FUNCTION FC 80 : VOID
TITLE =BLOCK FOR BALANCING PRESS
AUTHOR : Esposito
FAMILY : EGAL_srl
NAME : BALANCIN
VERSION : 0.1


VAR_TEMP
  VALUE_TONN : REAL ;	//Value in tonn of the weight slide addition die
  VALUE_BAR : REAL ;	//Value in Bar of the cylinders balancing slide
  OFF_SET_LOAD : REAL ;	//Value in Bar of the OFF SET for load valve balancing
  OFF_SET_DISC : REAL ;	//Value in Bar of the OFF SET for discarge valve balancing
  OFF_SET_LOAD_H : REAL ;
  OFF_SET_DISC_L : REAL ;
  TON_VIS_OP37 : REAL ;
  MIN_MAX_VAL_OP37 : REAL ;
END_VAR
BEGIN
NETWORK
TITLE =CONDITIONS FOR BALANCING
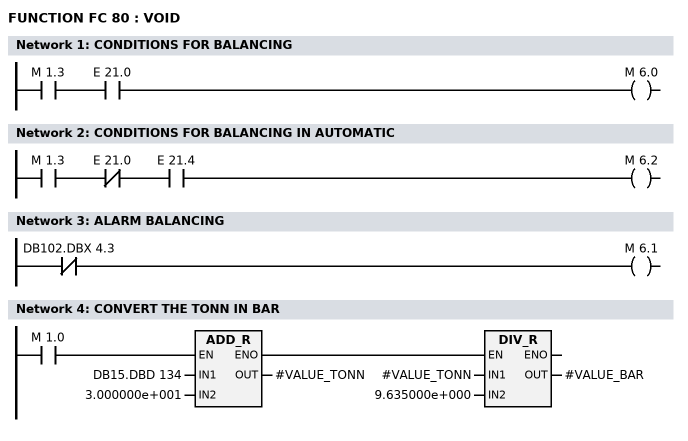
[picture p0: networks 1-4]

      U     M      1.3;
      U     E     21.0;
      =     M      6.0;
NETWORK
TITLE =CONDITIONS FOR BALANCING IN AUTOMATIC

      U     M      1.3;
      UN    E     21.0;
      U     E     21.4;
      =     M      6.2;
NETWORK
TITLE =ALARM BALANCING

      UN    DB102.DBX    4.3;
      =     M      6.1;
NETWORK
TITLE =CONVERT THE TONN IN BAR



      U(    ;
      U     M      1.0;
      SPBNB _018;
      L     DB15.DBD  134;
      L     3.000000e+001;
      +R    ;
      T     #VALUE_TONN;
      UN    OV;
      SAVE  ;
      CLR   ;
_018: U     BIE;
      )     ;
      SPBNB _019;
      L     #VALUE_TONN;
      L     9.635000e+000;
      /R    ;
      T     #VALUE_BAR;
_019: NOP   0;
NETWORK
TITLE =ENABLE/DISABLE AUTOMATIC BALANCING

      U(    ;
      U     M      1.0;
      U     M     47.1;
      S     M     48.0;
      U     M     47.2;
      R     M     48.0;
      U     M     48.0;
      )     ;
      NOT   ;
      =     M     48.1;
NETWORK
TITLE =CONTROL VALUE FOR COMAND THE ELECTRICAL VALVE
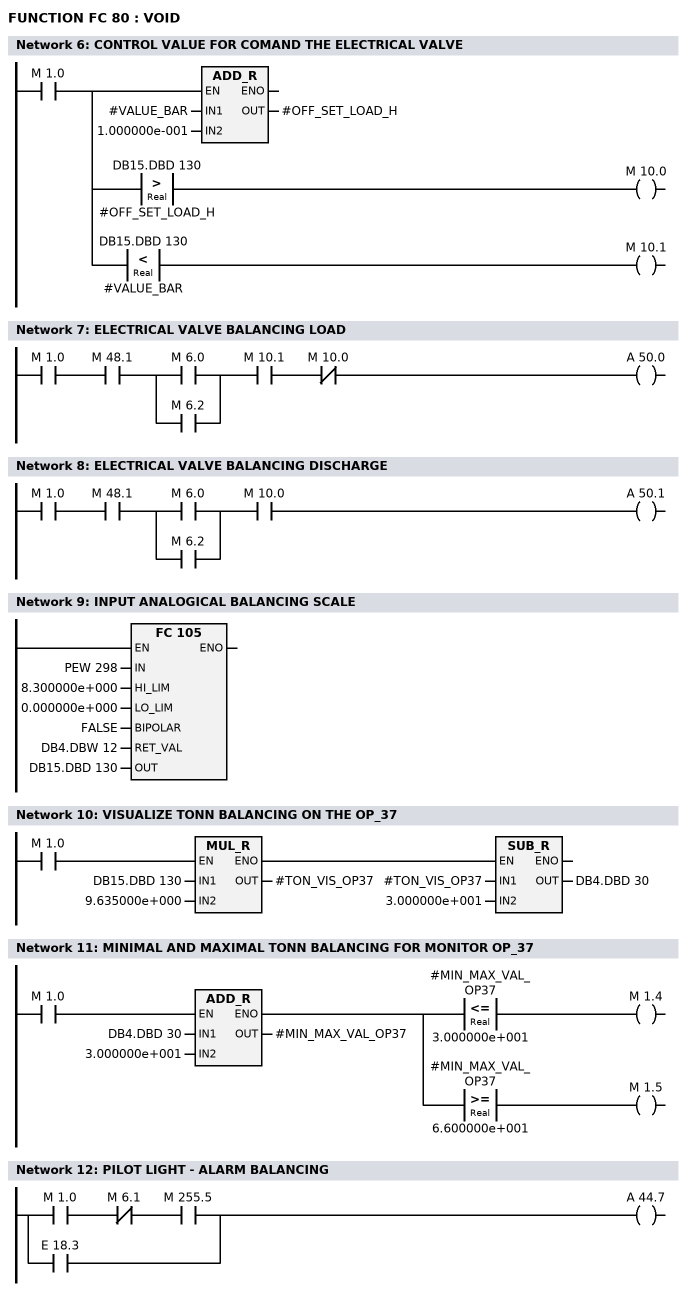
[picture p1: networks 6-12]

      U     M      1.0;
      =     L     32.0;
      U     L     32.0;
      SPBNB _01a;
      L     #VALUE_BAR;
      L     1.000000e-001;
      +R    ;
      T     #OFF_SET_LOAD_H;
_01a: NOP   0;
      U     L     32.0;
      U(    ;
      L     DB15.DBD  130;
      L     #OFF_SET_LOAD_H;
      >R    ;
      )     ;
      =     M     10.0;
      U     L     32.0;
      U(    ;
      L     DB15.DBD  130;
      L     #VALUE_BAR;
      <R    ;
      )     ;
      =     M     10.1;
NETWORK
TITLE =ELECTRICAL VALVE BALANCING LOAD

      U     M      1.0;
      U     M     48.1;
      U(    ;
      O     M      6.0;
      O     M      6.2;
      )     ;
      U     M     10.1;
      UN    M     10.0;
      =     A     50.0;
NETWORK
TITLE =ELECTRICAL VALVE BALANCING DISCHARGE

      U     M      1.0;
      U     M     48.1;
      U(    ;
      O     M      6.0;
      O     M      6.2;
      )     ;
      U     M     10.0;
      =     A     50.1;
NETWORK
TITLE =INPUT ANALOGICAL BALANCING SCALE

      CALL FC   105 (
           IN                       := PEW  298,
           HI_LIM                   := 8.300000e+000,
           LO_LIM                   := 0.000000e+000,
           BIPOLAR                  := FALSE,
           RET_VAL                  := DB4.DBW   12,
           OUT                      := DB15.DBD  130);


NETWORK
TITLE =VISUALIZE TONN BALANCING ON THE OP_37

      U(    ;
      U     M      1.0;
      SPBNB _01b;
      L     DB15.DBD  130;
      L     9.635000e+000;
      *R    ;
      T     #TON_VIS_OP37;
      UN    OV;
      SAVE  ;
      CLR   ;
_01b: U     BIE;
      )     ;
      SPBNB _01f;
      L     #TON_VIS_OP37;
      L     3.000000e+001;
      -R    ;
      T     DB4.DBD   30;
_01f: NOP   0;
NETWORK
TITLE =MINIMAL AND MAXIMAL TONN BALANCING FOR MONITOR OP_37

      U     M      1.0;
      SPBNB _020;
      L     DB4.DBD   30;
      L     3.000000e+001;
      +R    ;
      T     #MIN_MAX_VAL_OP37;
      UN    OV;
      SAVE  ;
      CLR   ;
_020: U     BIE;
      =     L     32.0;
      U     L     32.0;
      U(    ;
      L     #MIN_MAX_VAL_OP37;
      L     3.000000e+001;
      <=R   ;
      )     ;
      =     M      1.4;
      U     L     32.0;
      U(    ;
      L     #MIN_MAX_VAL_OP37;
      L     6.600000e+001;
      >=R   ;
      )     ;
      =     M      1.5;
NETWORK
TITLE =PILOT LIGHT - ALARM BALANCING

      U     M      1.0;
      UN    M      6.1;
      U     M    255.5;
      O     E     18.3;
      =     A     44.7;
END_FUNCTION

